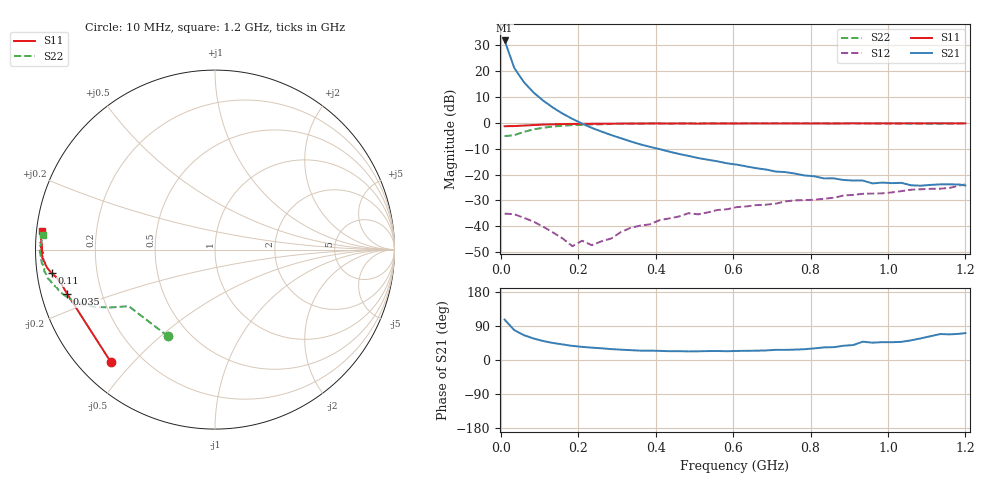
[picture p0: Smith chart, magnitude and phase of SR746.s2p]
!  POLYFET RF DEVICES
!  SR746
!  (Each side)
!  S PARAMETERS
!  VDS=50V, IDQ=400mA
# MHZ S MA R 50
! Freq=Mhz Mag[s11] Ang[s11] Mag[s21] Ang[s21] Mag[s12] Ang[s12] Mag[s22] Ang[s22]
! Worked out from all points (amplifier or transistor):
!   49 points, 10 MHz to 1.2 GHz, reference 50 ohm
!   highest |S21| = 31.7 dB at 10 MHz (marker M1)
!   |S21| within 3 dB of that: start of sweep to 17.05 MHz
!   unconditionally stable (mu >= 1): 172.8 MHz to 309.8 MHz; 346.2 MHz to 372.8 MHz; 549.2 MHz to end of sweep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
!   at 210 MHz: K = 1.05, MAG = 21.2 dB, |S12| = -45.5 dB
!   at 610 MHz: K = 1.01, MAG = 7.5 dB, |S12| = -32.6 dB
!   at 1.2 GHz: K = 1.43, MAG = -4.1 dB, |S12| = -23.8 dB
!   S11 on the Smith chart (normalised r, x): 10 MHz: 0.09, -0.43; 35 MHz: 0.08, -0.15; 110 MHz: 0.04, -0.07; 1.2 GHz: 0.02, +0.05
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10  0.8537 -132.9  38.54 106.5  0.01761 17.8  0.5495 -118.4
35  0.8596 -163.3  11.33 78.8  0.01716 -8.7  0.5749 -146.7
60  0.8807 -168.1  6.029 65.5  0.01459 -17.3  0.6652 -151.0
85  0.8993 -170.3  3.805 56.7  0.01234 -24.3  0.7431 -154.6
110  0.92 -171.8  2.648 50.0  0.00981 -25.4  0.7985 -157.7
135  0.9296 -172.7  1.951 44.9  0.00762 -24.9  0.8439 -160.4
160  0.939 -173.7  1.492 41.0  0.00583 -8.6  0.8725 -162.8
185  0.9479 -174.8  1.185 37.3  0.00415 14.9  0.8991 -165.1
210  0.9503 -175.5  0.9611 34.7  0.00529 24.2  0.9065 -166.5
235  0.9538 -176.1  0.7943 32.6  0.00434 42.9  0.9261 -168.0
285  0.9572 -176.8  0.5781 28.8  0.00583 75.4  0.9457 -170.3
310  0.9615 -176.9  0.5019 27.3  0.00774 73.5  0.9465 -171.2
410  0.9689 -178.7  0.3093 24.1  0.01315 93.5  0.9597 -174.0
485  0.966 -179.1  0.2285 22.7  0.01796 95.1  0.9688 -175.7
510  0.9579 -179.0  0.208 22.9  0.01705 96.1  0.9676 -176.3
610  0.9641 -179.8  0.1552 23.9  0.02355 99.7  0.9723 -177.6
810  0.9658 179.5  0.09248 30.7  0.03271 106.3  0.9738 178.8
960  0.9683 178.2  0.06739 45.7  0.0429 106.7  0.9661 176.6
1010  0.97 177.5  0.06818 47.0  0.04517 110.2  0.9634 176.4
1085  0.9704 175.3  0.06089 57.1  0.05195 109.1  0.9595 175.5
1160  0.971 175.5  0.0647 67.6  0.05545 115.3  0.9591 175.4
1200  0.9705 174.0  0.06131 71.0  0.0645 112.6  0.9642 175.2
